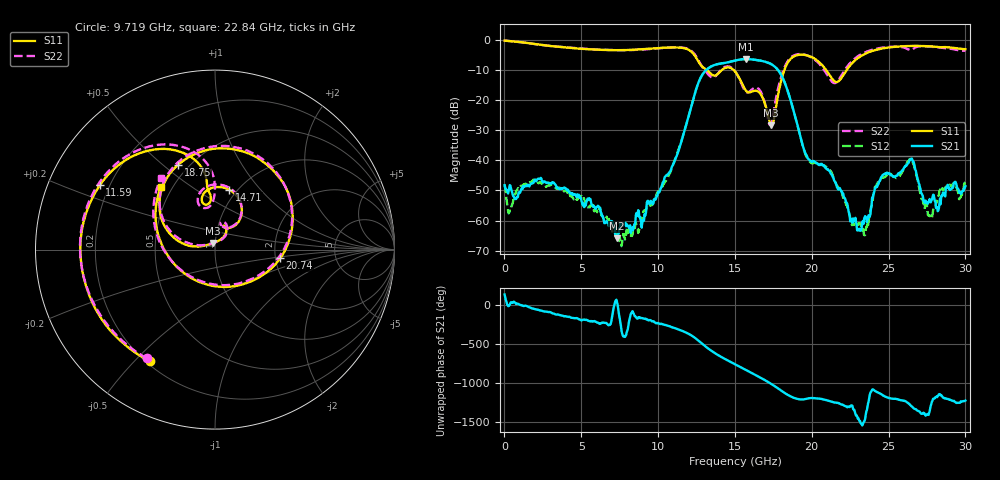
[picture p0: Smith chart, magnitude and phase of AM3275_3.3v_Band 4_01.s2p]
!Keysight Technologies,N5245B,MY58422270,A.16.20.02
!Date: Thursday, March 27, 2025 02:06:21
!Correction: S11(C  2-Port  )
!S21(C  2-Port  )
!S12(C  2-Port  )
!S22(C  2-Port  )
!S2P File: Measurements: S11, S21, S12, S22:
# Hz S  dB  R 50
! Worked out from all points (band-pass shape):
!   801 points, 10 MHz to 30 GHz, reference 50 ohm
!   highest |S21| = -6.37 dB at 15.72 GHz (marker M1); lowest = -66.0 dB at 7.32 GHz (marker M2)
!   |S21| within 3 dB of the highest: 13.28 GHz to 17.7 GHz (4.413 GHz wide, 28.5 % of centre)
!   lowest |S11| = -28.3 dB at 17.37 GHz (marker M3), VSWR 1.08, Z = 48.9 + j3.62 ohm
!   |S11| at or under -10 dB: 13.17 GHz to 14.15 GHz (982.1 MHz wide, 7.19 % of centre); 14.92 GHz to 18.22 GHz (3.3 GHz wide, 19.9 % of centre); 20.94 GHz to 22.27 GHz (1.338 GHz wide, 6.19 % of centre)
!   |S22| runs from -28.3 to -0.2 dB; largest |S21 - S12| = 0.0067
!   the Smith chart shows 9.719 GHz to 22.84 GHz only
!   S11 on the Smith chart (normalised r, x): 9.719 GHz: 0.21, -0.56; 11.59 GHz: 0.16, +0.25; 14.71 GHz: 0.92, +0.70; 18.75 GHz: 0.44, +0.56; 20.74 GHz: 2.12, -0.24; 22.84 GHz: 0.43, +0.38
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1e7  -0.24 -4.5  -48.26 131.1  -48.01 12.4  -0.19 -4.3
1.172112e9  -0.80 -82.1  -49.64 -6.7  -48.42 -9.3  -0.84 -82.1
2.521662e9  -1.75 -160.1  -47.34 -81.6  -47.53 -77.2  -1.74 -160.4
5.033325e9  -2.97 86.8  -53.82 160.5  -51.91 172.1  -2.87 86.0
7.320062e9  -3.42 -10.5  -65.97 38.3  -64.22 16.2  -3.41 -12.1
9.719262e9  -2.84 -120.2  -53.08 148.0  -53.66 140.2  -2.92 -122.0
1.001916e10  -2.73 -134.0  -50.49 119.3  -50.46 130.9  -2.80 -135.6
1.159364e10  -2.67 150.9  -32.33 24.1  -32.34 24.2  -2.56 149.9
1.324309e10  -10.31 94.8  -9.52 162.7  -9.52 162.5  -11.33 92.2
1.47051e10  -9.28 77.0  -7.26 -9.5  -7.25 -9.6  -9.01 77.8
1.5005e10  -10.47 62.1  -6.87 -39.9  -6.86 -40.0  -10.37 62.0
1.571726e10  -16.85 57.0  -6.37 -113.9  -6.36 -113.9  -17.26 63.3
1.646701e10  -17.03 65.7  -6.72 168.3  -6.73 168.2  -15.99 68.9
1.736671e10  -28.34 104.8  -8.06 67.1  -8.08 67.2  -27.73 128.1
1.875375e10  -5.75 113.5  -22.41 -104.4  -22.36 -103.8  -5.39 109.9
2.002832e10  -5.78 37.3  -40.54 -112.9  -40.99 -111.6  -6.00 33.5
2.074059e10  -8.73 -7.6  -41.65 -130.5  -41.66 -127.7  -9.53 -13.9
2.283989e10  -6.70 130.9  -59.12 46.4  -62.02 -17.6  -6.03 127.3
2.501416e10  -2.53 51.1  -44.40 -112.0  -44.48 -110.5  -2.31 48.9
2.647618e10  -2.02 11.0  -39.46 145.6  -39.64 146.4  -3.31 12.8
2.748834e10  -2.08 -17.7  -53.90 38.1  -54.56 -60.8  -2.18 -17.4
3e10  -3.07 -109.0  -48.60 -145.5  -47.39 -131.5  -3.58 -109.7
